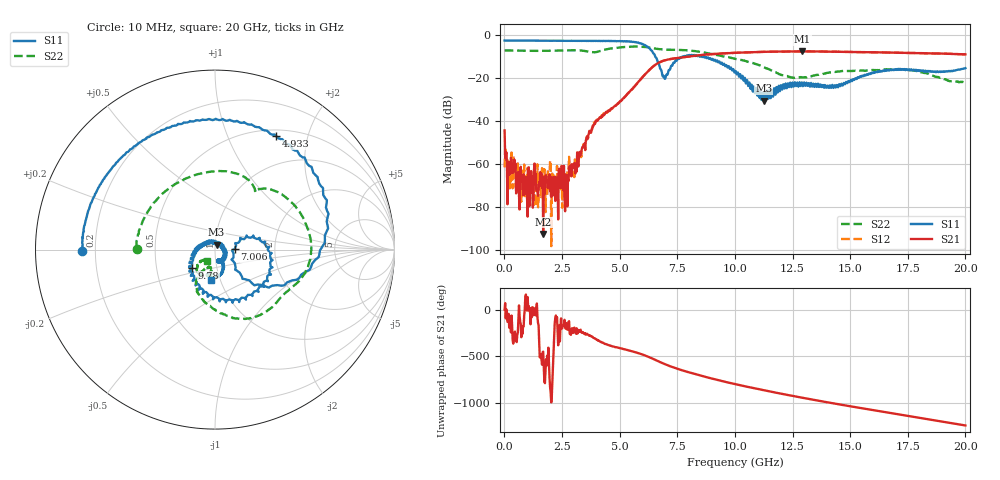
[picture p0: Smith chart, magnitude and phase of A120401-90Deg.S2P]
!  2-Port S-parameters saved by WinCal
! VAR MeasName=S-Parameters (CALIBRATED_DATA) read from VNA (N5244A)
! VAR MeasDate=11/21/2012 9:57:53 AM
! VAR NAME=A120401-90Deg
! VAR FILENAME=A120401-90Deg.S2P
! VAR DATE=11/21/2012 9:57:53 AM
! VAR PHYS_PORTS=1,2
# Hz S MA R 50
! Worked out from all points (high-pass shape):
!   801 points, 10 MHz to 20 GHz, reference 50 ohm
!   highest |S21| = -7.65 dB at 12.93 GHz (marker M1); lowest = -92.4 dB at 1.684 GHz (marker M2)
!   |S21| within 3 dB of the highest: 7.569 GHz to end of sweep
!   lowest |S11| = -30.6 dB at 11.25 GHz (marker M3), VSWR 1.06, Z = 50.8 + j2.86 ohm
!   |S11| at or under -10 dB: 6.545 GHz to 7.731 GHz (1.185 GHz wide, 16.6 % of centre); 7.734 GHz to 7.808 GHz (74 MHz wide, 0.952 % of centre); 8.646 GHz to end of sweep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
!   |S22| runs from -22.0 to -5.4 dB; largest |S21 - S12| = 0.0069
!   S11 on the Smith chart (normalised r, x): 10 MHz: 0.15, -0.00; 4.933 GHz: 0.58, +1.52; 7.006 GHz: 1.25, +0.01; 9.78 GHz: 0.76, -0.16; 20 GHz: 0.90, -0.31
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1e7  0.7429 -179.6  0.006048 0.8  0.0008341 166.9  0.4367 179.4
1.59925e8  0.7412 176.9  0.001103 -125.0  0.0009488 -125.3  0.4394 173.7
5.847125e8  0.7385 168.8  0.000638 116.8  0.001035 58.1  0.4324 157.7
1.384312e9  0.7356 153.1  0.0002526 2.1  0.000104 -64.6  0.4276 130.2
1.684162e9  0.7332 147.2  2.391e-05 -88.3  0.0005185 89.8  0.4267 120.2
2.233888e9  0.7315 135.8  0.0004932 -63.5  0.000339 -146.5  0.4307 102.2
2.483762e9  0.7317 130.4  0.0008891 163.0  0.0009097 -75.5  0.4351 93.9
2.70865e9  0.7297 125.7  0.0005577 155.4  0.0002809 62.9  0.4382 86.8
3.358325e9  0.7252 109.9  0.002249 122.0  0.002105 96.9  0.432 65.7
3.958025e9  0.7244 93.9  0.009944 48.9  0.009678 42.3  0.3981 55.3
4.932538e9  0.7181 61.6  0.02594 -46.3  0.02638 -47.6  0.509 28.3
5.90705e9  0.6412 10.6  0.09269 -112.1  0.09263 -111.7  0.5331 -4.6
6.681662e9  0.2233 -46.8  0.2238 168.7  0.2249 168.8  0.4705 -28.3
7.0065e9  0.1097 1.8  0.2613 133.7  0.2618 133.7  0.4549 -35.0
8.030988e9  0.3418 -24.1  0.3161 49.1  0.3167 49.2  0.4358 -60.7
9.780112e9  0.1629 -142.2  0.3785 -61.8  0.3778 -61.9  0.2976 -101.2
1.0005e10  0.1413 -161.0  0.3838 -74.3  0.3837 -74.3  0.2788 -105.4
1.125438e10  0.02956 72.2  0.4051 -139.8  0.4045 -139.8  0.1767 -121.3
1.292854e10  0.07143 -59.4  0.4146 140.3  0.4136 140.1  0.1026 -103.9
1.335332e10  0.06272 -70.1  0.413 121.0  0.4132 120.8  0.1118 -103.0
1.667666e10  0.1505 -84.0  0.3904 -20.0  0.3896 -20.2  0.1587 -119.8
2e10  0.1687 -98.1  0.3538 -155.3  0.3545 -155.5  0.08086 -124.9
